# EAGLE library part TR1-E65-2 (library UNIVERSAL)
Trafo E65 s prehodenymi vyvodami.
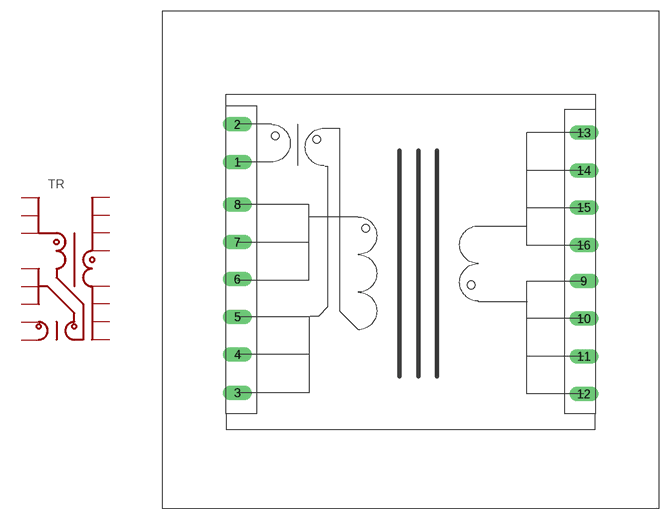
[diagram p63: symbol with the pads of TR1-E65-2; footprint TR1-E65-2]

Designator prefix TR

## TR1-E65-2  [TR1-E65-2]
1  1
2  2
3  3
4  4
5  5
6  6
7  7
8  8
9  9
10  10
11  11
12  12
13  13
14  14
15  15
16  16

## Footprint TR1-E65-2 (pad centres in mm)
drill 0.8 pad 1.93 long: 1 10,-20.06; 2 10,-15.06; 3 10,-50.7; 4 10,-45.62; 5 10,-40.62; 6 10,-35.62; 7 10,-30.7; 8 10,-25.7; 9 56,-35.86; 10 56,-40.86; 11 56,-45.86; 12 56,-50.86; 13 56,-16.172; 14 56,-21.172; 15 56,-26.093; 16 56,-31.093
